FUNCTION_BLOCK Example33_StarWheelSetup	//Initial setup for Example33_StarWheel
VAR_INPUT
	Execute : BOOL;
END_VAR
VAR_OUTPUT
	Done : BOOL;
END_VAR
VAR_IN_OUT
	PM_Controller : PMControllerType;	// the planar motor controller to use
END_VAR
VAR
	PMC_StopXbots1 : PMC_StopXbots;
	PMC_DeleteStarWheel1 : PMC_Star_DeleteStar;
	PMC_ClearMacro1 : PMC_ClearMacro;
	PMC_XYMotion1 : PMC_XYMotion;
	PMC_ArcMotionTarget1 : PMC_ArcMotionTarget;
	PMC_XYMotion2 : PMC_XYMotion;
	PMC_ArcMotionTarget2 : PMC_ArcMotionTarget;
	PMC_XYMotion3 : PMC_XYMotion;
	PMC_SaveMacro1 : PMC_SaveMacro;
	PMC_AutoDrivingMotion1 : PMC_AutoDrivingMotion;
	XbotIDs : ARRAY[0..77] OF USINT;
	PosXs : ARRAY[0..77] OF REAL;
	PosYs : ARRAY[0..77] OF REAL;
	PMC_XYMotion4 : PMC_XYMotion;
	xbot_id : USINT := 1;
	PMC_CreateStarWheel1 : PMC_Star_CreateStar;
	Vials : ARRAY[0..99] OF REAL;
	PMC_StreamModeCtrl1 : PMC_StreamModeCtrl;	
	Disc_Radius : REAL := 0.3;
	Disc_X : REAL := 0.36;
	Disc_Y : REAL := 0.36;
	Clearance_Space : REAL := 0.15;
END_VAR

VAR CONSTANT
	PI : REAL := 3.141593;
	
END_VAR

//Initial setup for Example33_StarWheel

//Reset xbot ID
IF(NOT(Execute))THEN
	xbot_id := 1;
END_IF;

//Stop all xbots
PMC_StopXbots1(Execute := Execute,XbotID := 0,PM_Controller := PM_Controller);

//Delete all star wheels
PMC_DeleteStarWheel1(Execute := PMC_StopXbots1.Done,WheelID := 0,PM_Controller := PM_Controller);

//setup star wheel module
Vials[0] := 0;Vials[1] := PI/2;Vials[2] := PI;Vials[3] := 3*PI/2;
PMC_CreateStarWheel1(Execute := PMC_DeleteStarWheel1.Done,WheelID := 1,Direction := 1,MasterXID := 100,DiscRadius := Disc_Radius,MaxDiscSpeed := 5,MaxXbotAcc := 10,DiscCenterX := Disc_X,
					DiscCenterY := Disc_Y,StartX := Disc_X + Disc_Radius,StartY := 0.06,EndX := Disc_X - Clearance_Space,EndY := Disc_Y + Disc_Radius,SyncStart := 0,SyncEnd := PI/2,NumVials := 4,VialLocations := Vials,PM_Controller := PM_Controller);

//Setup macro 128
PMC_ClearMacro1(Execute := PMC_CreateStarWheel1.Done,MacroID := 128,PM_Controller := PM_Controller);
PMC_XYMotion1(Execute := PMC_ClearMacro1.Done,cmdLB := 0,XbotID := 128,Mode := 0,Type_ := 0,PosX := 0.18,PosY := Disc_Y + Disc_Radius,EndVel := 1,MaxVel := 1,MaxAcc := 20,PM_Controller := PM_Controller);
PMC_ArcMotionTarget1(Execute := PMC_XYMotion1.Done,cmdLB := 0,XbotID := 128,Mode := 0,AType := 0,Dir := 1,EndVel := 1,MaxVel := 1,MaxAcc := 20,PosX := 0.06,PosY := PMC_XYMotion1.PosY - 0.12,Radius := 0.12,PM_Controller := PM_Controller);
PMC_XYMotion2(Execute := PMC_ArcMotionTarget1.Done,cmdLB := 0,XbotID := 128,Mode := 0,Type_ := 0,PosX := 0.06,PosY := 0.18,EndVel := 1,MaxVel := 1,MaxAcc := 20,PM_Controller := PM_Controller);
PMC_ArcMotionTarget2(Execute := PMC_XYMotion2.Done,cmdLB := 0,XbotID := 128,Mode := 0,AType := 0,Dir := 1,EndVel := 1,MaxVel := 1,MaxAcc := 20,PosX := 0.18,PosY := 0.06,Radius := 0.12,PM_Controller := PM_Controller);
PMC_XYMotion3(Execute := PMC_ArcMotionTarget2.Done,cmdLB := 0,XbotID := 128,Mode := 0,Type_ := 0,PosX := Disc_X + Disc_Radius,PosY := 0.06,EndVel := 0,MaxVel := 2,MaxAcc := 20,PM_Controller := PM_Controller);
PMC_SaveMacro1(Execute := PMC_XYMotion3.Done,MacroID := 128,PM_Controller := PM_Controller);

//Move xbots to starting positions
XbotIDs[0] := 1;XbotIDs[1] := 2;XbotIDs[2] := 3;XbotIDs[3] := 4;XbotIDs[4] := 5;XbotIDs[5] := 6;
PosXs[0] := 0.06;PosXs[1] := 0.06;PosXs[2] := 0.06;PosXs[3] := 0.06;PosXs[4] := 0.06;PosXs[5] := 0.06;
PosYs[0] := 0.06;PosYs[1] := 0.18;PosYs[2] := 0.30;PosYs[3] := 0.42;PosYs[4] := 0.54;PosYs[5] := 0.66;
PMC_AutoDrivingMotion1(Execute := PMC_SaveMacro1.Done,nXbots := 6,RoutingType := 0,ZoneID := 0,XbotID := XbotIDs,PosX := PosXs,PosY := PosYs,PM_Controller := PM_Controller);

//setup xbot queueing
PMC_XYMotion4(Execute := PMC_AutoDrivingMotion1.Done,cmdLB := 0,XbotID := xbot_id,Mode := 0,Type_ := 2,PosX := Disc_X + Disc_Radius,PosY := 0.06,EndVel := 0,MaxVel := 2,MaxAcc := 20,PM_Controller := PM_Controller);
IF(PMC_XYMotion4.Ack AND xbot_id < 6)THEN
	PMC_XYMotion4(Execute := FALSE,PM_Controller := PM_Controller);
	xbot_id := xbot_id + 1;
END_IF;

//setup streaming to virtual xbot 100
PMC_StreamModeCtrl1.XbotID[0] := 100;
PMC_StreamModeCtrl1.StmID[0] := 1;
PMC_StreamModeCtrl1.StmAxis[0] := 32;
PMC_StreamModeCtrl1.offsetX[0] := 0;
PMC_StreamModeCtrl1.offsetY[0] := 0;
PMC_StreamModeCtrl1(Execute := PMC_XYMotion4.Ack,Level := 1,nXbots := 1,PM_Controller := PM_Controller);
Done := PMC_StreamModeCtrl1.Done;

END_FUNCTION_BLOCK
